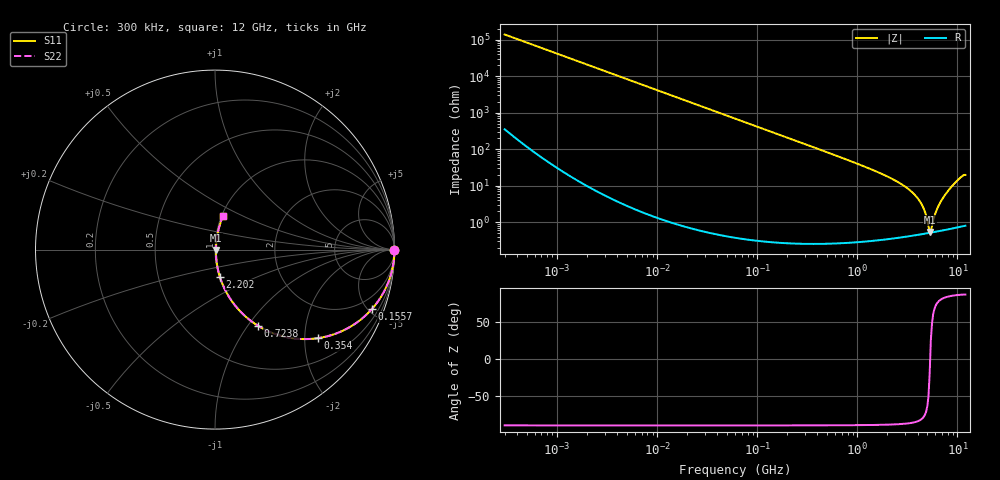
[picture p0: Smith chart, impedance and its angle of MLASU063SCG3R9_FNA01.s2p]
! MLASU063SCG3R9_FNA01  S-PARAMETER MODEL  ( Standard Model )
! Model Generated by TAIYO YUDEN Corporation (http://www.ty-top.com)
! Version 1.0
! TAIYO YUDEN Control No. 240819
! Copyright(c) 2024 TAIYO YUDEN CO.,LTD. All Rights Reserved.
! Product Description (link to TY-COMPAS)
! https://ds.yuden.co.jp/TYCOMPAS/or/detail?pn=MLASU063SCG3R9CFNA01&u=M
! Products Name : Multilayer Ceramic Capacitors
! Characteristics :
!  Capacitance : 3.9 [pF] , Rated Voltage : 50 [V] , TCC : CG / C0G
!  Case Size : 0.6 x 0.3 / 0.024 x 0.012 [mm/inch] , Thickness : 0.3 / 0.012 [mm/inch]
!  (Conditions: Temperature = 25 [degC] , DC Bias Voltage = 0 [V])
! External Node Assignments :
!  1  o---| |---o  2
! GND o---------o GND
! Frequency Range : 0.3MHz  -  12000MHz  [ 401 STEP ]
# MHZ S RI R 50
! Freq[MHz].  S11 Real  S11 Imag  S21 Real  S21 Imag  S12 Real  S12 Imag  S22 Real  S22 Imag
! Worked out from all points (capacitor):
!   401 points, 300 kHz to 12 GHz, reference 50 ohm
!   read as one part in series: C = 3.85 pF near 316.3 kHz
!   lowest |Z| = 539 mohm at 5.279 GHz (marker M1)
!   series resonance near 5.337 GHz, so ESL is about 230 pH
!   S11 on the Smith chart (normalised r, x): 300 kHz: open; 155.7 MHz: 1.01, -5.30; 354 MHz: 1.01, -2.32; 723.8 MHz: 1.01, -1.12; 2.202 GHz: 1.01, -0.31; 12 GHz: 1.02, +0.39
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0.3  1 -0.000726  2.38e-06 0.000726  2.38e-06 0.000726  1 -0.000726
1.769972  1 -0.00429  2.05e-05 0.00429  2.05e-05 0.00429  1 -0.00429
10.44266  0.9994 -0.0253  0.000647 0.0253  0.000647 0.0253  0.9994 -0.0253
60  0.9793 -0.1423  0.0207 0.1423  0.0207 0.1423  0.9793 -0.1423
155.7172  0.8751 -0.3301  0.1249 0.3301  0.1249 0.3301  0.8751 -0.3301
353.9943  0.5742 -0.4934  0.4258 0.4934  0.4258 0.4934  0.5742 -0.4934
723.8279  0.2399 -0.4246  0.7601 0.4246  0.7601 0.4246  0.2399 -0.4246
1166.079  0.1042 -0.3012  0.8958 0.3012  0.8958 0.3012  0.1042 -0.3012
2088.533  0.0305 -0.1618  0.9695 0.1618  0.9695 0.1618  0.0305 -0.1618
2202.174  0.0269 -0.1509  0.9731 0.1509  0.9731 0.1509  0.0269 -0.1509
3107.553  0.0116 -0.0865  0.9884 0.0865  0.9884 0.0865  0.0116 -0.0865
3944.255  0.00666 -0.047  0.9933 0.047  0.9933 0.047  0.00666 -0.047
4502.883  0.0054 -0.0262  0.9946 0.0262  0.9946 0.0262  0.0054 -0.0262
4747.894  0.00515 -0.018  0.9948 0.018  0.9948 0.018  0.00515 -0.018
5140.631  0.00505 -0.00577  0.995 0.00577  0.995 0.00577  0.00505 -0.00577
5278.635  0.00508 -0.00172  0.9949 0.00172  0.9949 0.00172  0.00508 -0.00172
5565.855  0.00525 0.00583  0.9948 -0.00583  0.9948 -0.00583  0.00525 0.00583
6026.253  0.00571 0.0167  0.9943 -0.0167  0.9943 -0.0167  0.00571 0.0167
6354.153  0.00617 0.0244  0.9938 -0.0244  0.9938 -0.0244  0.00617 0.0244
7448.838  0.00888 0.0529  0.9911 -0.0529  0.9911 -0.0529  0.00888 0.0529
9708.23  0.0229 0.1248  0.9771 -0.1248  0.9771 -0.1248  0.0229 0.1248
12000  0.0443 0.1864  0.9557 -0.1864  0.9557 -0.1864  0.0443 0.1864
